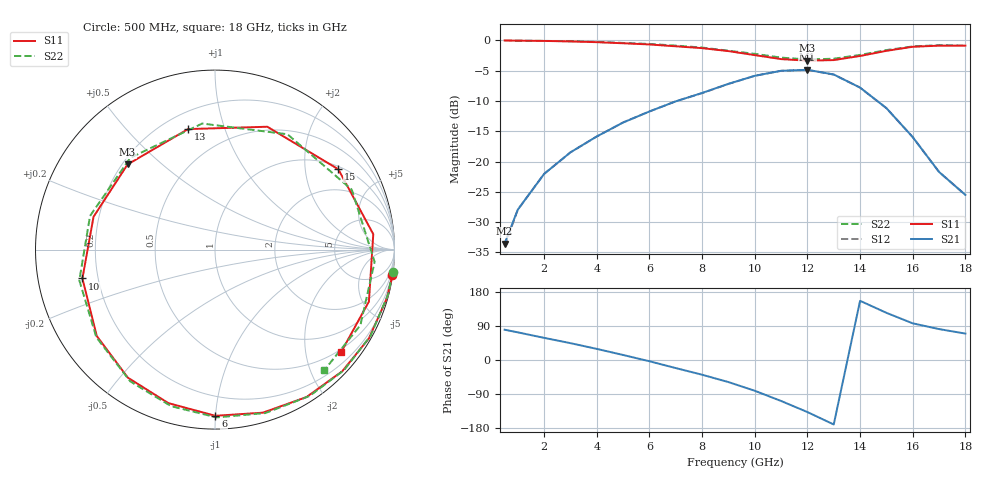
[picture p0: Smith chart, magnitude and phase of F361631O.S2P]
!ATF-36163
!VDS=0 VGS=-1.5V
! last updated 11-10-95
# ghz s ma r 50
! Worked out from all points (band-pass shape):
!   19 points, 500 MHz to 18 GHz, reference 50 ohm
!   highest |S21| = -4.85 dB at 12 GHz (marker M1); lowest = -33.6 dB at 500 MHz (marker M2)
!   |S21| within 3 dB of the highest: 8.549 GHz to 14.02 GHz (5.47 GHz wide, 48.5 % of centre)
!   lowest |S11| = -3.3 dB at 12 GHz (marker M3), VSWR 5.25, Z = 11 + j19.5 ohm
!   |S11| at or under -10 dB: nowhere
!   |S22| runs from -3.1 to 0.0 dB; largest |S21 - S12| = 0.0025
!   S11 on the Smith chart (normalised r, x): 500 MHz: 0, -14; 6 GHz: 0.08, -1.00; 10 GHz: 0.14, -0.11; 13 GHz: 0.30, +0.76; 15 GHz: 1.10, +3.00; 18 GHz: 0.44, -2.77
0.5  0.999 -8.2  0.021 79.9  0.02 80.1  0.998 -7.2
1  0.995 -15.8  0.04 73.0  0.04 72.9  0.996 -14.6
2  0.99 -29.9  0.079 58.4  0.079 58.6  0.991 -29.0
3  0.981 -43.7  0.119 44.5  0.119 44.5  0.984 -43.1
4  0.967 -58.1  0.161 29.3  0.161 29.4  0.971 -57.1
5  0.947 -73.6  0.21 13.3  0.21 13.4  0.953 -72.9
6  0.926 -89.9  0.259 -3.3  0.259 -3.1  0.935 -89.5
7  0.894 -106.9  0.314 -21.3  0.314 -21.1  0.906 -105.6
8  0.863 -124.2  0.368 -38.9  0.367 -38.7  0.873 -122.7
9  0.816 -143.8  0.438 -58.2  0.437 -58.1  0.822 -143.5
10  0.756 -167.7  0.51 -81.2  0.51 -81.0  0.775 -167.2
11  0.701 164.9  0.561 -108.1  0.561 -107.9  0.721 164.9
12  0.68 135.8  0.572 -137.4  0.571 -137.2  0.696 132.7
13  0.688 102.6  0.523 -170.2  0.522 -169.9  0.706 95.8
14  0.744 66.9  0.408 156.1  0.407 156.3  0.759 57.8
15  0.82 33.1  0.276 124.5  0.276 124.7  0.832 23.7
16  0.886 5.6  0.159 96.7  0.159 97.0  0.892 -4.4
17  0.905 -18.6  0.082 81.6  0.082 81.7  0.913 -27.4
18  0.905 -38.9  0.053 69.7  0.053 70.2  0.907 -47.8
